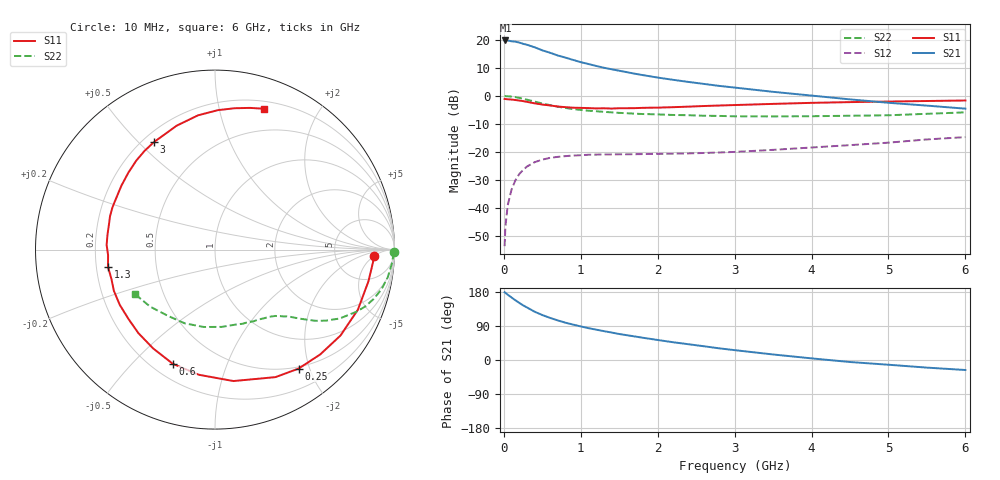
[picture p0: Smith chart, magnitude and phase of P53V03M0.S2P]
! SIEMENS Small Signal Semiconductors
! BFP183
! Si NPN RF Bipolar Junction Transistor in SOT143
! VCE = 3 V  IC = 3 mA
! Common Emitter S-Parameters:  March  1996
# GHz  S  MA  R  50
!  f  S11  S21  S12  S22
! GHz  MAG  ANG  MAG  ANG  MAG  ANG  MAG  ANG
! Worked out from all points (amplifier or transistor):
!   36 points, 10 MHz to 6 GHz, reference 50 ohm
!   highest |S21| = 19.8 dB at 20 MHz (marker M1)
!   |S21| within 3 dB of that: start of sweep to 452.2 MHz
!   unconditionally stable (mu >= 1): 1.889 GHz to 5.806 GHz
!   at 250 MHz: K = 0.15, MSG = 22.5 dB, |S12| = -26.4 dB
!   at 1.4 GHz: K = 0.79, MSG = 15.2 dB, |S12| = -20.8 dB
!   at 6 GHz: K = 0.97, MSG = 5.1 dB, |S12| = -14.7 dB
!   lowest NFmin = 1.10 dB at 450 MHz
!   S11 on the Smith chart (normalised r, x): 10 MHz: 15, -5; 250 MHz: 0.47, -1.83; 600 MHz: 0.28, -0.66; 1.3 GHz: 0.25, -0.08; 3 GHz: 0.24, +0.56; 6 GHz: 0.27, +1.37
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0.01  0.8845 -2.2  9.676 178.7  0.0021 86.7  0.9961 -0.9
0.02  0.8829 -4.7  9.769 177.5  0.0046 79.8  0.9939 -1.9
0.05  0.8729 -11.7  9.764 172.4  0.0112 84.1  0.9882 -4.6
0.15  0.8474 -34.4  9.289 157.6  0.0313 71.4  0.9529 -13.5
0.2  0.8275 -44.9  8.966 150.8  0.0405 66.2  0.9255 -17.3
0.25  0.8101 -54.9  8.515 144.3  0.048 61.0  0.8941 -20.8
0.3  0.7865 -64.6  8.204 138.7  0.0551 56.3  0.8595 -23.8
0.4  0.7396 -82.0  7.379 127.5  0.066 48.3  0.794 -28.9
0.5  0.7032 -97.3  6.517 118.6  0.0733 41.9  0.7347 -32.6
0.6  0.6786 -110.2  5.899 111.2  0.0788 37.0  0.6867 -35.3
0.7  0.6496 -122.0  5.279 104.5  0.0821 33.2  0.6447 -37.3
0.8  0.6315 -132.5  4.828 98.5  0.0846 30.2  0.6118 -39.0
0.9  0.618 -141.1  4.398 93.5  0.0868 27.5  0.5842 -40.5
1.1  0.6084 -157.8  3.712 84.0  0.0896 23.6  0.5465 -42.9
1.3  0.604 -170.8  3.188 76.2  0.0909 21.2  0.5208 -45.4
1.6  0.6048 172.1  2.657 65.4  0.0913 19.1  0.4922 -49.0
2.2  0.6314 145.7  1.942 46.9  0.0935 19.7  0.4585 -58.2
3  0.6888 119.6  1.412 26.0  0.1006 23.1  0.4341 -73.7
3.5  0.7226 107.2  1.186 14.6  0.1095 24.9  0.4323 -85.0
4.5  0.7772 88.8  0.87 -5.3  0.133 25.3  0.4441 -112.3
5.5  0.8133 76.1  0.673 -20.1  0.168 22.9  0.481 -138.6
6  0.8313 70.7  0.594 -26.4  0.1847 19.3  0.5106 -151.0
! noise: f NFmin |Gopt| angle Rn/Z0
0.45  1.1  0.37  35  0.3
0.9  1.15  0.34  85  0.23
1.8  1.9  0.35  160  0.13
